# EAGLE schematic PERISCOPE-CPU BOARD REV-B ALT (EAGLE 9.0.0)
This Set of Many Schematics Is what comprises the Revision-B PCB, of my eden project "PERISCOPE". (CPU BOARD ONLY)

## Sheet 1 of 10: Clock, Horizontal Sync
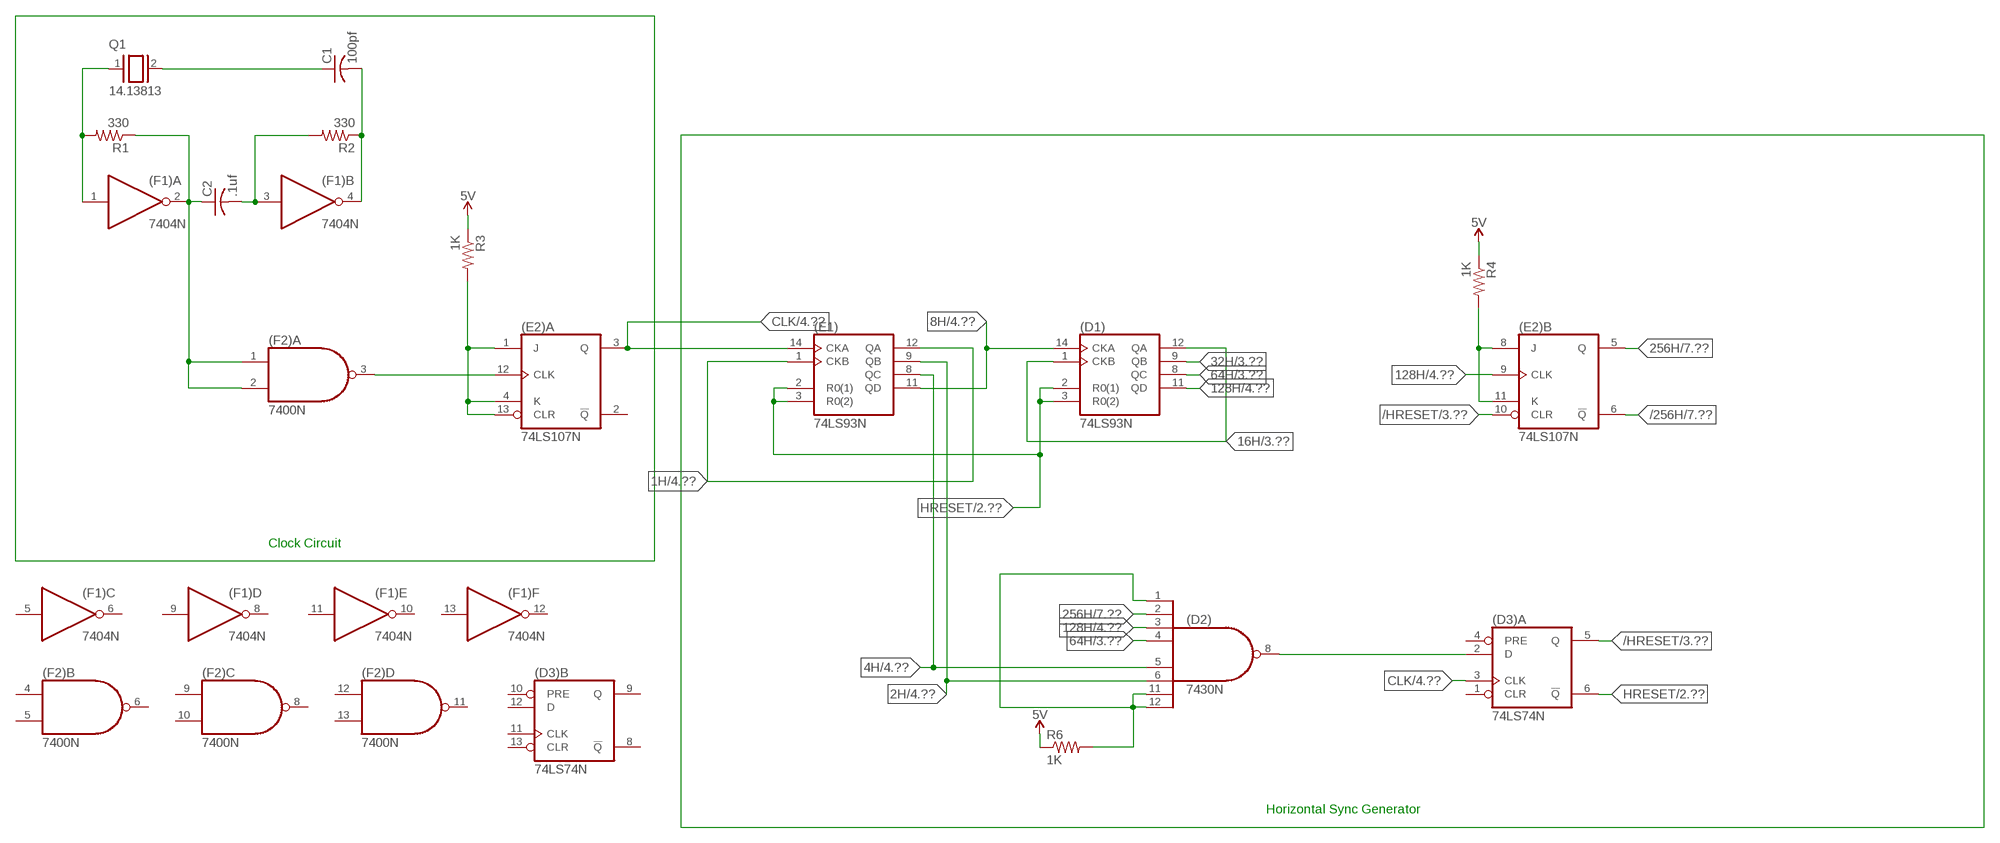
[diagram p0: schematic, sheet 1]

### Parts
(D1)  74LS93N  [DIL14]
(D2)  7430N  [DIL14]
(D3)  74LS74N  [DIL14]
(E1)  74LS93N  [DIL14]
(E2)  74LS107N  [DIL14]
(F1)  7404N  [DIL14]
(F2)  7400N  [DIL14]
C1  100pf  C-US050-025X075  [C050-025X075]
C2  .1uf  C-US050-025X075  [C050-025X075]
Q1  14.13813  XTAL/S  [QS]
R1  330  R-US_0207/10  [0207/10]
R2  330  R-US_0207/10  [0207/10]
R3  1K  R-US_0207/10  [0207/10]
R4  1K  R-US_0207/10  [0207/10]
R6  1K  R-US_0207/10  [0207/10]

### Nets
1H: (E1).1(CKB) (E1).12(QA) ; also sheet 4,8
2H: (D2).6(I5) (E1).9(QB) ; also sheet 4,5,8
4H: (D2).5(I4) (E1).8(QC) ; also sheet 4,7,8
5V: R3.1 R4.1 R6.1 ; also sheet 2
8H: (D1).14(CKA) (E1).11(QD) ; also sheet 4,7,8
16H: (D1).1(CKB) (D1).12(QA) ; also sheet 3,4,7,8
32H: (D1).9(QB) ; also sheet 3,4,7,8
64H: (D1).8(QC) (D2).4(I3) ; also sheet 3,4,7,8
128H: (D1).11(QD) (D2).3(I2) (E2).9(B:CLK) ; also sheet 4,7,8
256H: (D2).2(I1) (E2).5(B:Q) ; also sheet 7,8
512H: (D2).1(I0) (D2).11(I6) (D2).12(I7) R6.2
/256H: (E2).6(B:!Q) ; also sheet 7,8
/HRESET: (D3).5(A:Q) (E2).10(B:CLR) ; also sheet 3,8
CLK: (D3).3(A:CLK) (E1).14(CKA) (E2).3(A:Q) ; also sheet 4,8
HRESET: (D1).2(R0(1)) (D1).3(R0(2)) (D3).6(A:!Q) (E1).2(R0(1)) (E1).3(R0(2)) ; also sheet 2,8
N$1: C1.1 Q1.2
N$2: (F1).4(B:O) C1.2 R2.1
N$3: (F1).2(A:O) (F2).1(A:I0) (F2).2(A:I1) C2.1 R1.1
N$4: (F1).3(B:I) C2.2 R2.2
N$5: (F1).1(A:I) Q1.1 R1.2
N$6: (E2).12(A:CLK) (F2).3(A:O)
N$7: (E2).1(A:J) (E2).4(A:K) (E2).13(A:CLR) R3.2
N$8: (E2).8(B:J) (E2).11(B:K) R4.2
N$11: (D2).8(O) (D3).2(A:D)
Unconnected: (D3).1(A:CLR) (D3).4(A:PRE) (D3).8(B:!Q) (D3).9(B:Q) (D3).10(B:PRE) (D3).11(B:CLK) (D3).12(B:D) (D3).13(B:CLR) (E2).2(A:!Q) (F1).5(C:I) (F1).6(C:O) (F1).8(D:O) (F1).9(D:I) (F1).10(E:O) (F1).11(E:I) (F1).12(F:O) (F1).13(F:I) (F2).4(B:I0) (F2).5(B:I1) (F2).6(B:O) (F2).8(C:O) (F2).9(C:I0) (F2).10(C:I1) (F2).11(D:O) (F2).12(D:I0) (F2).13(D:I1)

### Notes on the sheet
- Clock Circuit
- Horizontal Sync Generator

## Sheet 2 of 10: Vertical Sync Generator
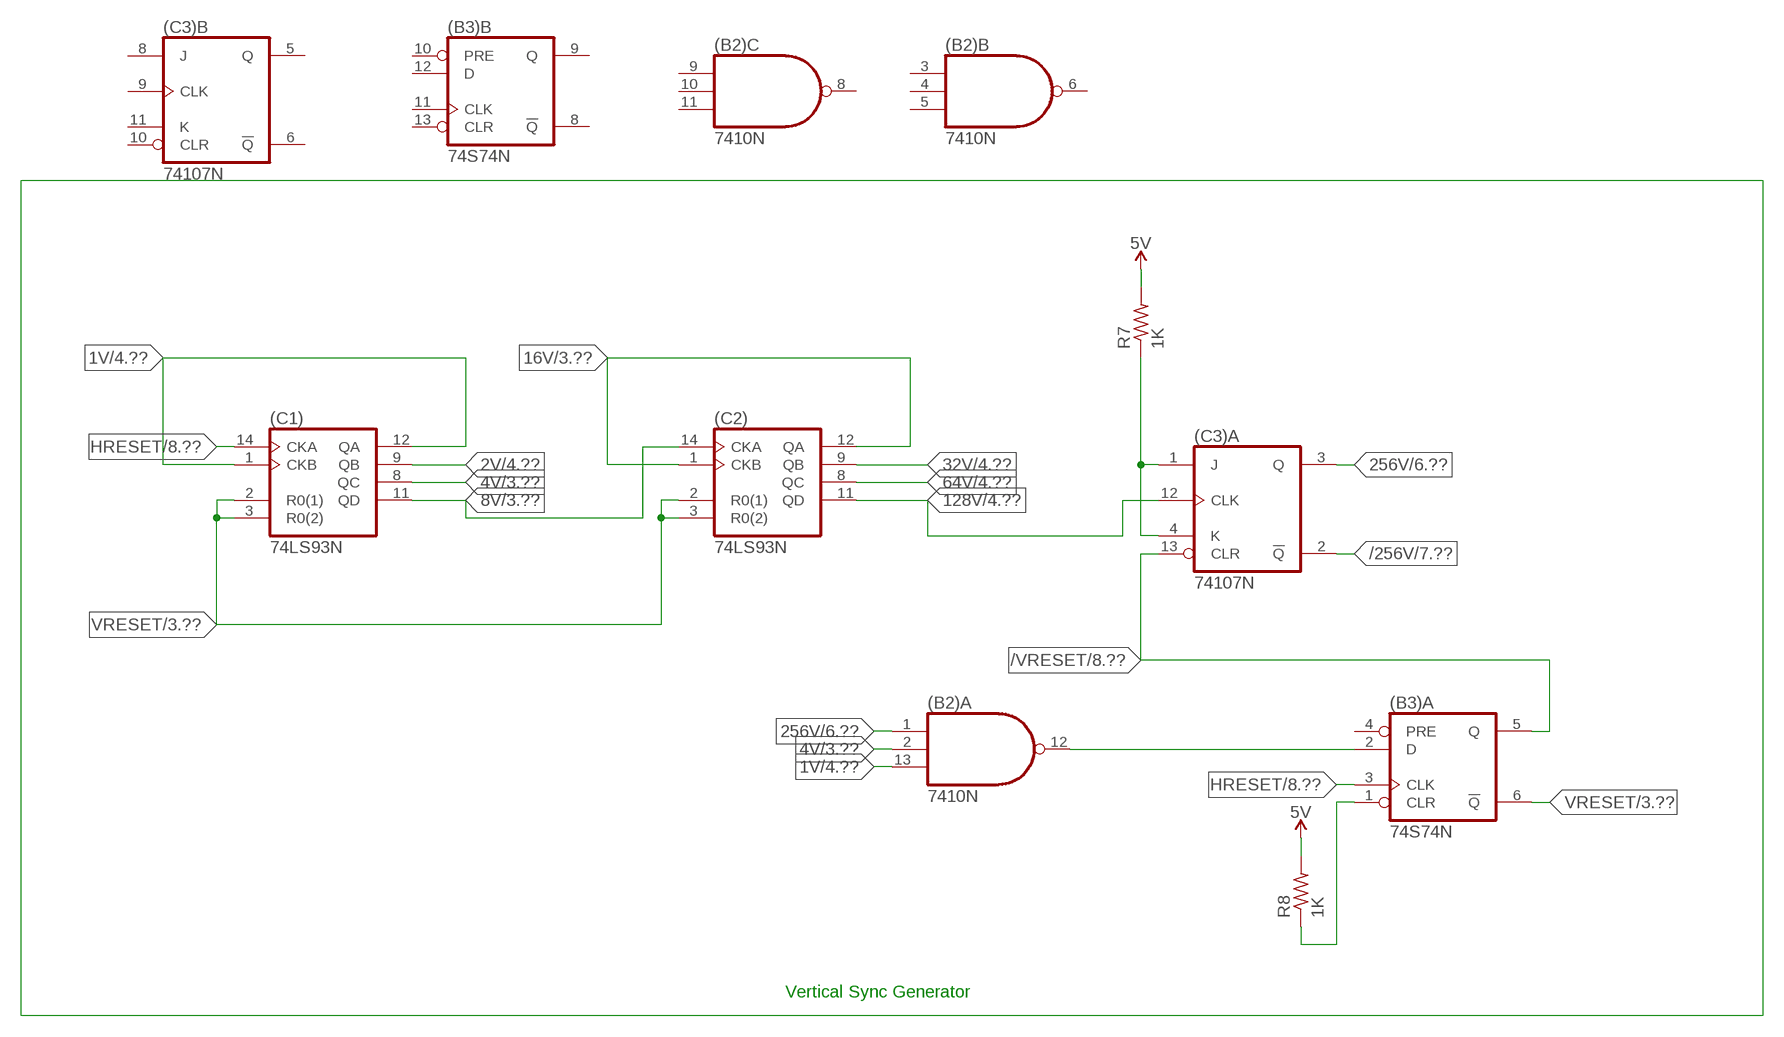
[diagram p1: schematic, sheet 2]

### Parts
(B2)  7410N  [DIL14]
(B3)  74S74N  [DIL14]
(C1)  74LS93N  [DIL14]
(C2)  74LS93N  [DIL14]
(C3)  74107N  [DIL14]
R7  1K  R-US_0207/10  [0207/10]
R8  1K  R-US_0207/10  [0207/10]

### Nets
1V: (B2).13(A:I2) (C1).1(CKB) (C1).12(QA) ; also sheet 4,8
2V: (C1).9(QB) ; also sheet 4,8
4V: (B2).2(A:I1) (C1).8(QC) ; also sheet 3,4,7,8
5V: R7.2 R8.2 ; also sheet 1
8V: (C1).11(QD) (C2).14(CKA) ; also sheet 3,4,7,8
16V: (C2).1(CKB) (C2).12(QA) ; also sheet 3,4,7,8
32V: (C2).9(QB) ; also sheet 4,7,8
64V: (C2).8(QC) ; also sheet 4,8
128V: (C2).11(QD) (C3).12(A:CLK) ; also sheet 4,5,6,8
256V: (B2).1(A:I0) (C3).3(A:Q) ; also sheet 6,8
/256V: (C3).2(A:!Q) ; also sheet 7,8
/VRESET: (B3).5(A:Q) (C3).13(A:CLR) ; also sheet 8
HRESET: (B3).3(A:CLK) (C1).14(CKA) ; also sheet 1,8
N$15: (C3).1(A:J) (C3).4(A:K) R7.1
N$16: (B3).1(A:CLR) R8.1
N$17: (B2).12(A:O) (B3).2(A:D)
VRESET: (B3).6(A:!Q) (C1).2(R0(1)) (C1).3(R0(2)) (C2).2(R0(1)) (C2).3(R0(2)) ; also sheet 3,8
Unconnected: (B2).3(B:I0) (B2).4(B:I1) (B2).5(B:I2) (B2).6(B:O) (B2).8(C:O) (B2).9(C:I0) (B2).10(C:I1) (B2).11(C:I2) (B3).4(A:PRE) (B3).8(B:!Q) (B3).9(B:Q) (B3).10(B:PRE) (B3).11(B:CLK) (B3).12(B:D) (B3).13(B:CLR) (C3).5(B:Q) (C3).6(B:!Q) (C3).8(B:J) (C3).9(B:CLK) (C3).10(B:CLR) (C3).11(B:K)

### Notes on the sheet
- Vertical Sync Generator

## Sheet 3 of 10: Sync Generation
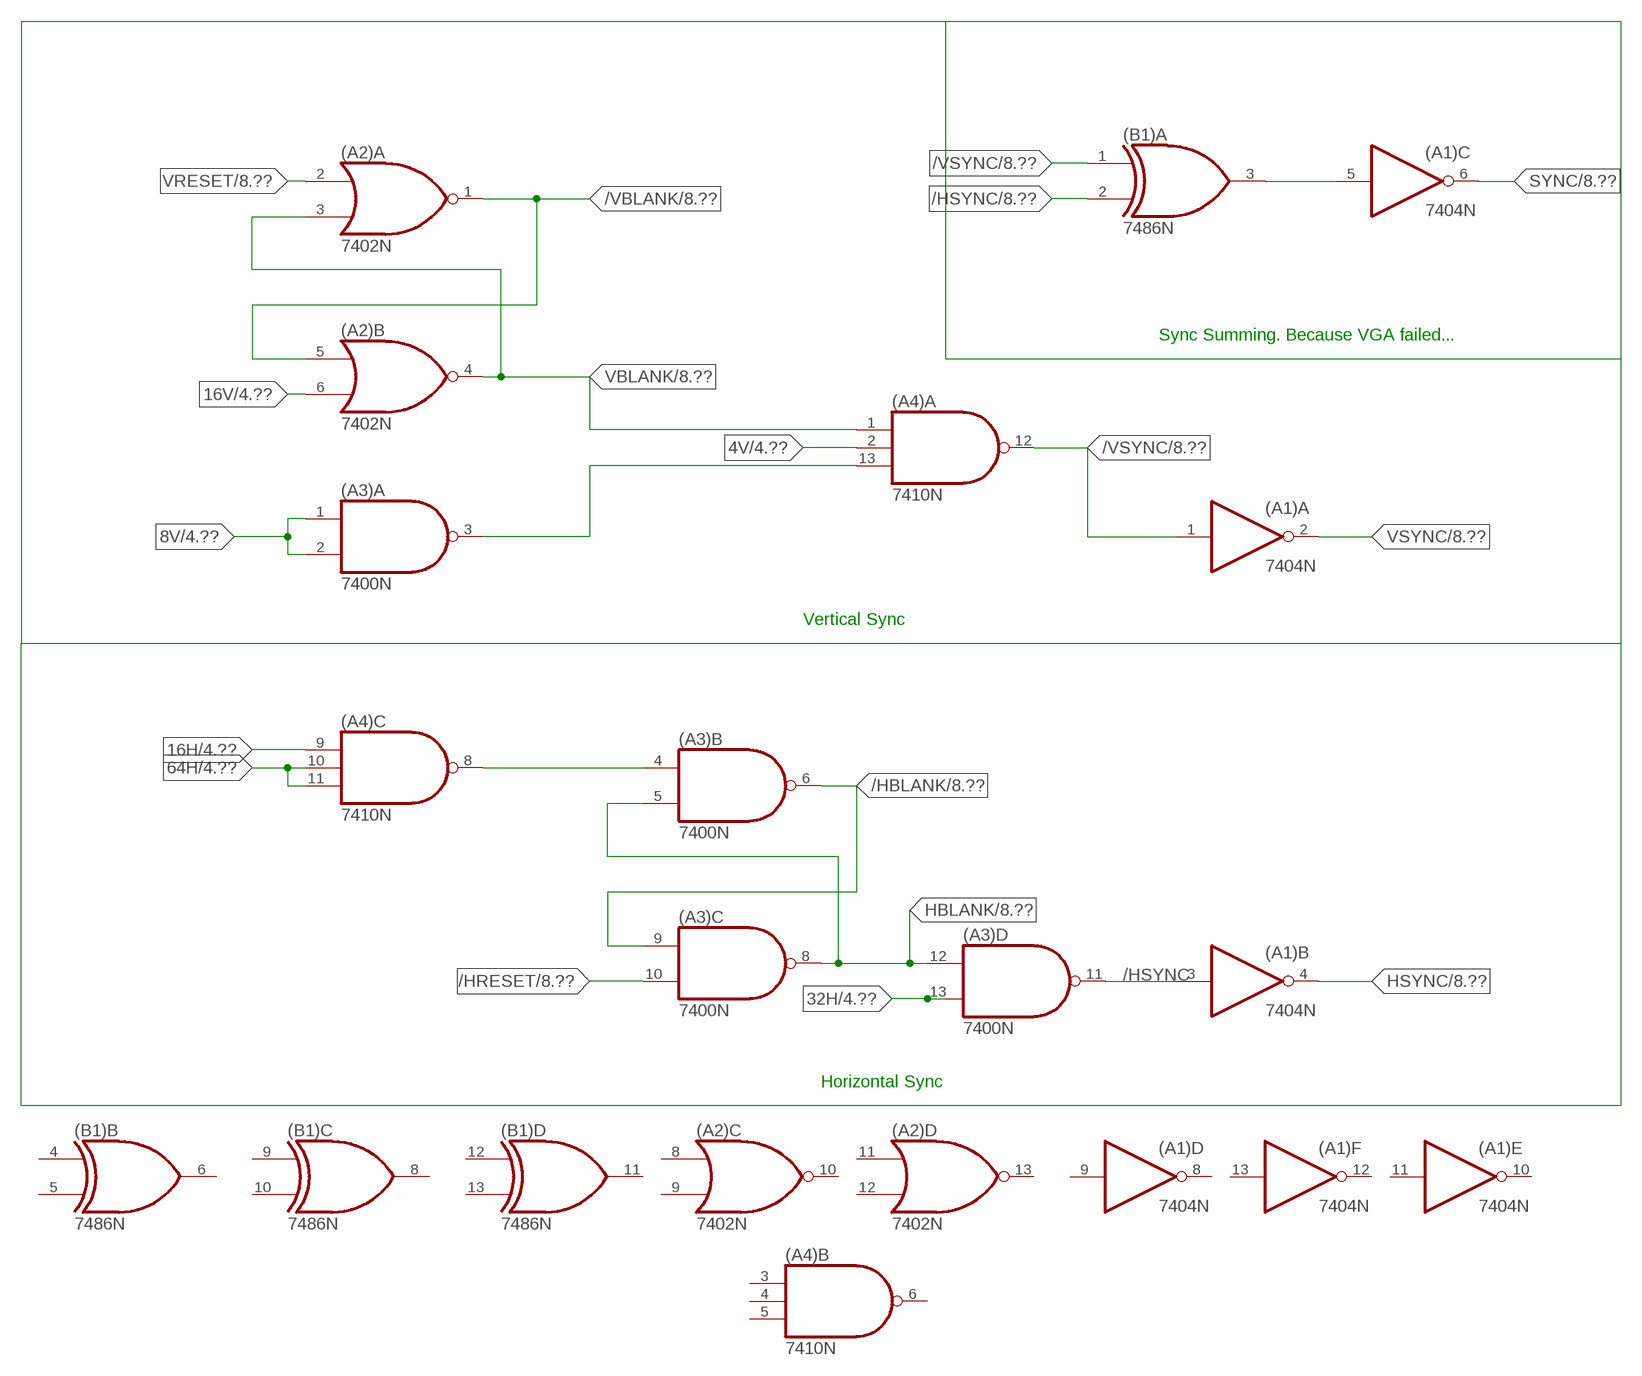
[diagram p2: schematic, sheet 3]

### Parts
(A1)  7404N  [DIL14]
(A2)  7402N  [DIL14]
(A3)  7400N  [DIL14]
(A4)  7410N  [DIL14]
(B1)  7486N  [DIL14]

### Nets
4V: (A4).2(A:I1) ; also sheet 2,4,7,8
8V: (A3).1(A:I0) (A3).2(A:I1) ; also sheet 2,4,7,8
16H: (A4).9(C:I0) ; also sheet 1,4,7,8
16V: (A2).6(B:I1) ; also sheet 2,4,7,8
32H: (A3).13(D:I1) ; also sheet 1,4,7,8
64H: (A4).10(C:I1) (A4).11(C:I2) ; also sheet 1,4,7,8
/HBLANK: (A3).6(B:O) (A3).9(C:I0) ; also sheet 8
/HRESET: (A3).10(C:I1) ; also sheet 1,8
/HSYNC: (A1).3(B:I) (A3).11(D:O) (B1).2(A:I1) ; also sheet 8
/VBLANK: (A2).1(A:O) (A2).5(B:I0) ; also sheet 8
/VSYNC: (A1).1(A:I) (A4).12(A:O) (B1).1(A:I0) ; also sheet 8
HBLANK: (A3).5(B:I1) (A3).8(C:O) (A3).12(D:I0) ; also sheet 8
HSYNC: (A1).4(B:O) ; also sheet 8
N$19: (A3).4(B:I0) (A4).8(C:O)
N$20: (A3).3(A:O) (A4).13(A:I2)
N$22: (A1).5(C:I) (B1).3(A:O)
SYNC: (A1).6(C:O) ; also sheet 8,10
VBLANK: (A2).3(A:I1) (A2).4(B:O) (A4).1(A:I0) ; also sheet 8
VRESET: (A2).2(A:I0) ; also sheet 2,8
VSYNC: (A1).2(A:O) ; also sheet 8
Unconnected: (A1).8(D:O) (A1).9(D:I) (A1).10(E:O) (A1).11(E:I) (A1).12(F:O) (A1).13(F:I) (A2).8(C:I0) (A2).9(C:I1) (A2).10(C:O) (A2).11(D:I0) (A2).12(D:I1) (A2).13(D:O) (A4).3(B:I0) (A4).4(B:I1) (A4).5(B:I2) (A4).6(B:O) (B1).4(B:I0) (B1).5(B:I1) (B1).6(B:O) (B1).8(C:O) (B1).9(C:I0) (B1).10(C:I1) (B1).11(D:O) (B1).12(D:I0) (B1).13(D:I1)

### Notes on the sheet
- Sync Summing. Because VGA failed...
- Vertical Sync
- Horizontal Sync

## Sheet 4 of 10: SYNC INVERSION
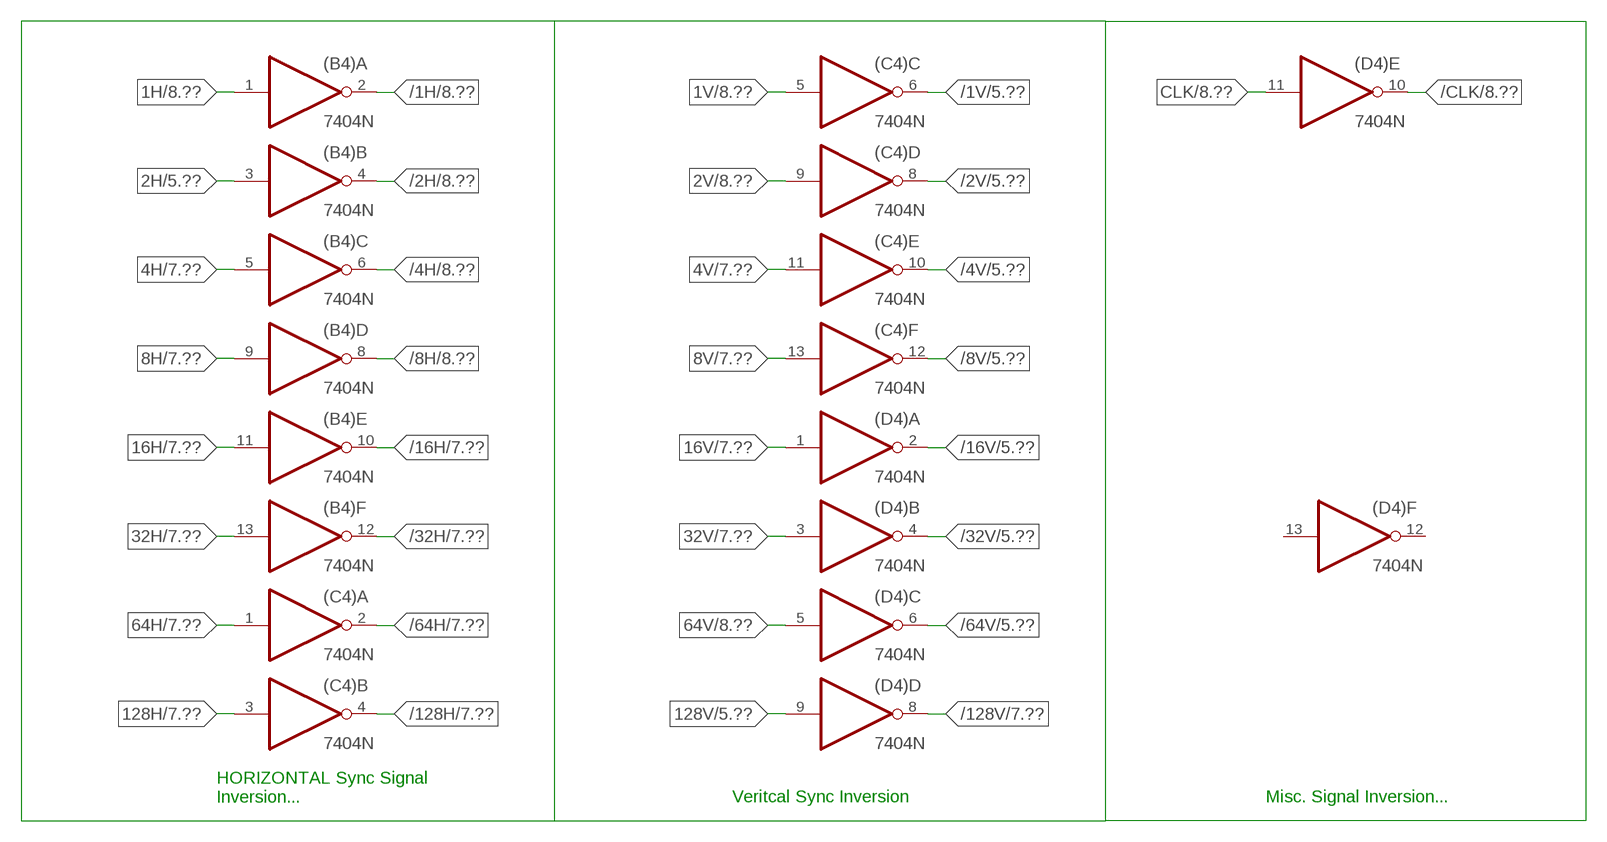
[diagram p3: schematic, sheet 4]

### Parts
(B4)  7404N  [DIL14]
(C4)  7404N  [DIL14]
(D4)  7404N  [DIL14]

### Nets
1H: (B4).1(A:I) ; also sheet 1,8
1V: (C4).5(C:I) ; also sheet 2,8
2H: (B4).3(B:I) ; also sheet 1,5,8
2V: (C4).9(D:I) ; also sheet 2,8
4H: (B4).5(C:I) ; also sheet 1,7,8
4V: (C4).11(E:I) ; also sheet 2,3,7,8
8H: (B4).9(D:I) ; also sheet 1,7,8
8V: (C4).13(F:I) ; also sheet 2,3,7,8
16H: (B4).11(E:I) ; also sheet 1,3,7,8
16V: (D4).1(A:I) ; also sheet 2,3,7,8
32H: (B4).13(F:I) ; also sheet 1,3,7,8
32V: (D4).3(B:I) ; also sheet 2,7,8
64H: (C4).1(A:I) ; also sheet 1,3,7,8
64V: (D4).5(C:I) ; also sheet 2,8
128H: (C4).3(B:I) ; also sheet 1,7,8
128V: (D4).9(D:I) ; also sheet 2,5,6,8
/1H: (B4).2(A:O) ; also sheet 8
/1V: (C4).6(C:O) ; also sheet 5,8
/2H: (B4).4(B:O) ; also sheet 8
/2V: (C4).8(D:O) ; also sheet 5,8
/4H: (B4).6(C:O) ; also sheet 8
/4V: (C4).10(E:O) ; also sheet 5,8
/8H: (B4).8(D:O) ; also sheet 8
/8V: (C4).12(F:O) ; also sheet 5,8
/16H: (B4).10(E:O) ; also sheet 7,8
/16V: (D4).2(A:O) ; also sheet 5,7,8
/32H: (B4).12(F:O) ; also sheet 7,8
/32V: (D4).4(B:O) ; also sheet 5,8
/64H: (C4).2(A:O) ; also sheet 7,8
/64V: (D4).6(C:O) ; also sheet 5,7,8
/128H: (C4).4(B:O) ; also sheet 7,8
/128V: (D4).8(D:O) ; also sheet 7,8
/CLK: (D4).10(E:O) ; also sheet 8
CLK: (D4).11(E:I) ; also sheet 1,8
Unconnected: (D4).12(F:O) (D4).13(F:I)

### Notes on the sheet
- HORIZONTAL Sync Signal
  Inversion...
- Veritcal Sync Inversion | Misc. Signal Inversion...

## Sheet 5 of 10: Ocean Generation, Surface and Floor
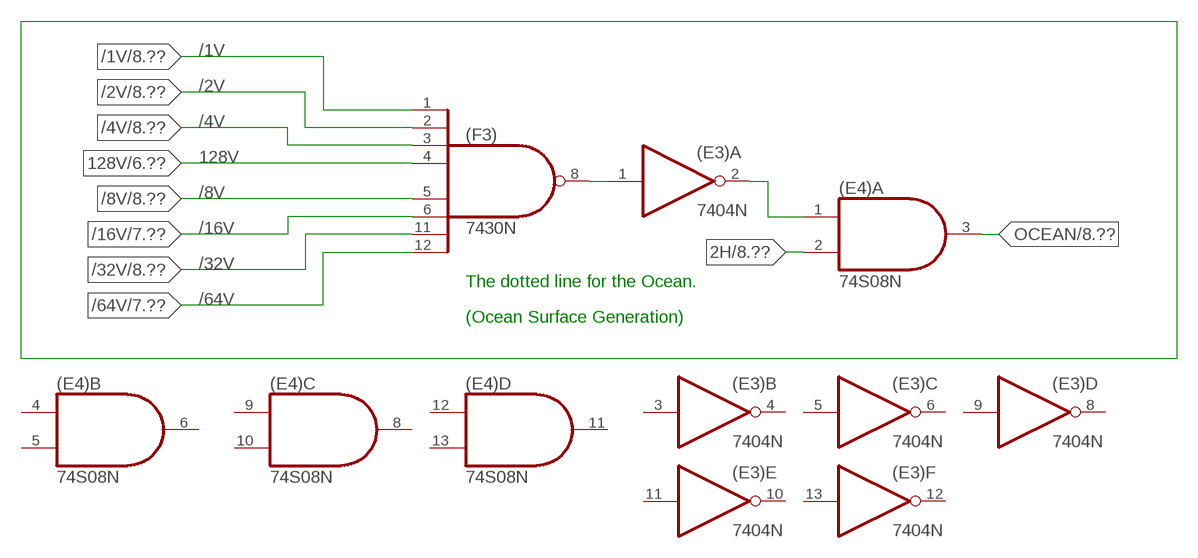
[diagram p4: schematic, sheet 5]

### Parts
(E3)  7404N  [DIL14]
(E4)  74S08N  [DIL14]
(F3)  7430N  [DIL14]

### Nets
2H: (E4).2(A:I1) ; also sheet 1,4,8
128V: (F3).4(I3) ; also sheet 2,4,6,8
/1V: (F3).1(I0) ; also sheet 4,8
/2V: (F3).2(I1) ; also sheet 4,8
/4V: (F3).3(I2) ; also sheet 4,8
/8V: (F3).5(I4) ; also sheet 4,8
/16V: (F3).6(I5) ; also sheet 4,7,8
/32V: (F3).11(I6) ; also sheet 4,8
/64V: (F3).12(I7) ; also sheet 4,7,8
N$28: (E3).1(A:I) (F3).8(O)
N$29: (E3).2(A:O) (E4).1(A:I0)
OCEAN: (E4).3(A:O) ; also sheet 8,9
Unconnected: (E3).3(B:I) (E3).4(B:O) (E3).5(C:I) (E3).6(C:O) (E3).8(D:O) (E3).9(D:I) (E3).10(E:O) (E3).11(E:I) (E3).12(F:O) (E3).13(F:I) (E4).4(B:I0) (E4).5(B:I1) (E4).6(B:O) (E4).8(C:O) (E4).9(C:I0) (E4).10(C:I1) (E4).11(D:O) (E4).12(D:I0) (E4).13(D:I1)

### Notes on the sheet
- The dotted line for the Ocean.
- (Ocean Surface Generation)

## Sheet 6 of 10: Coin Circuitry
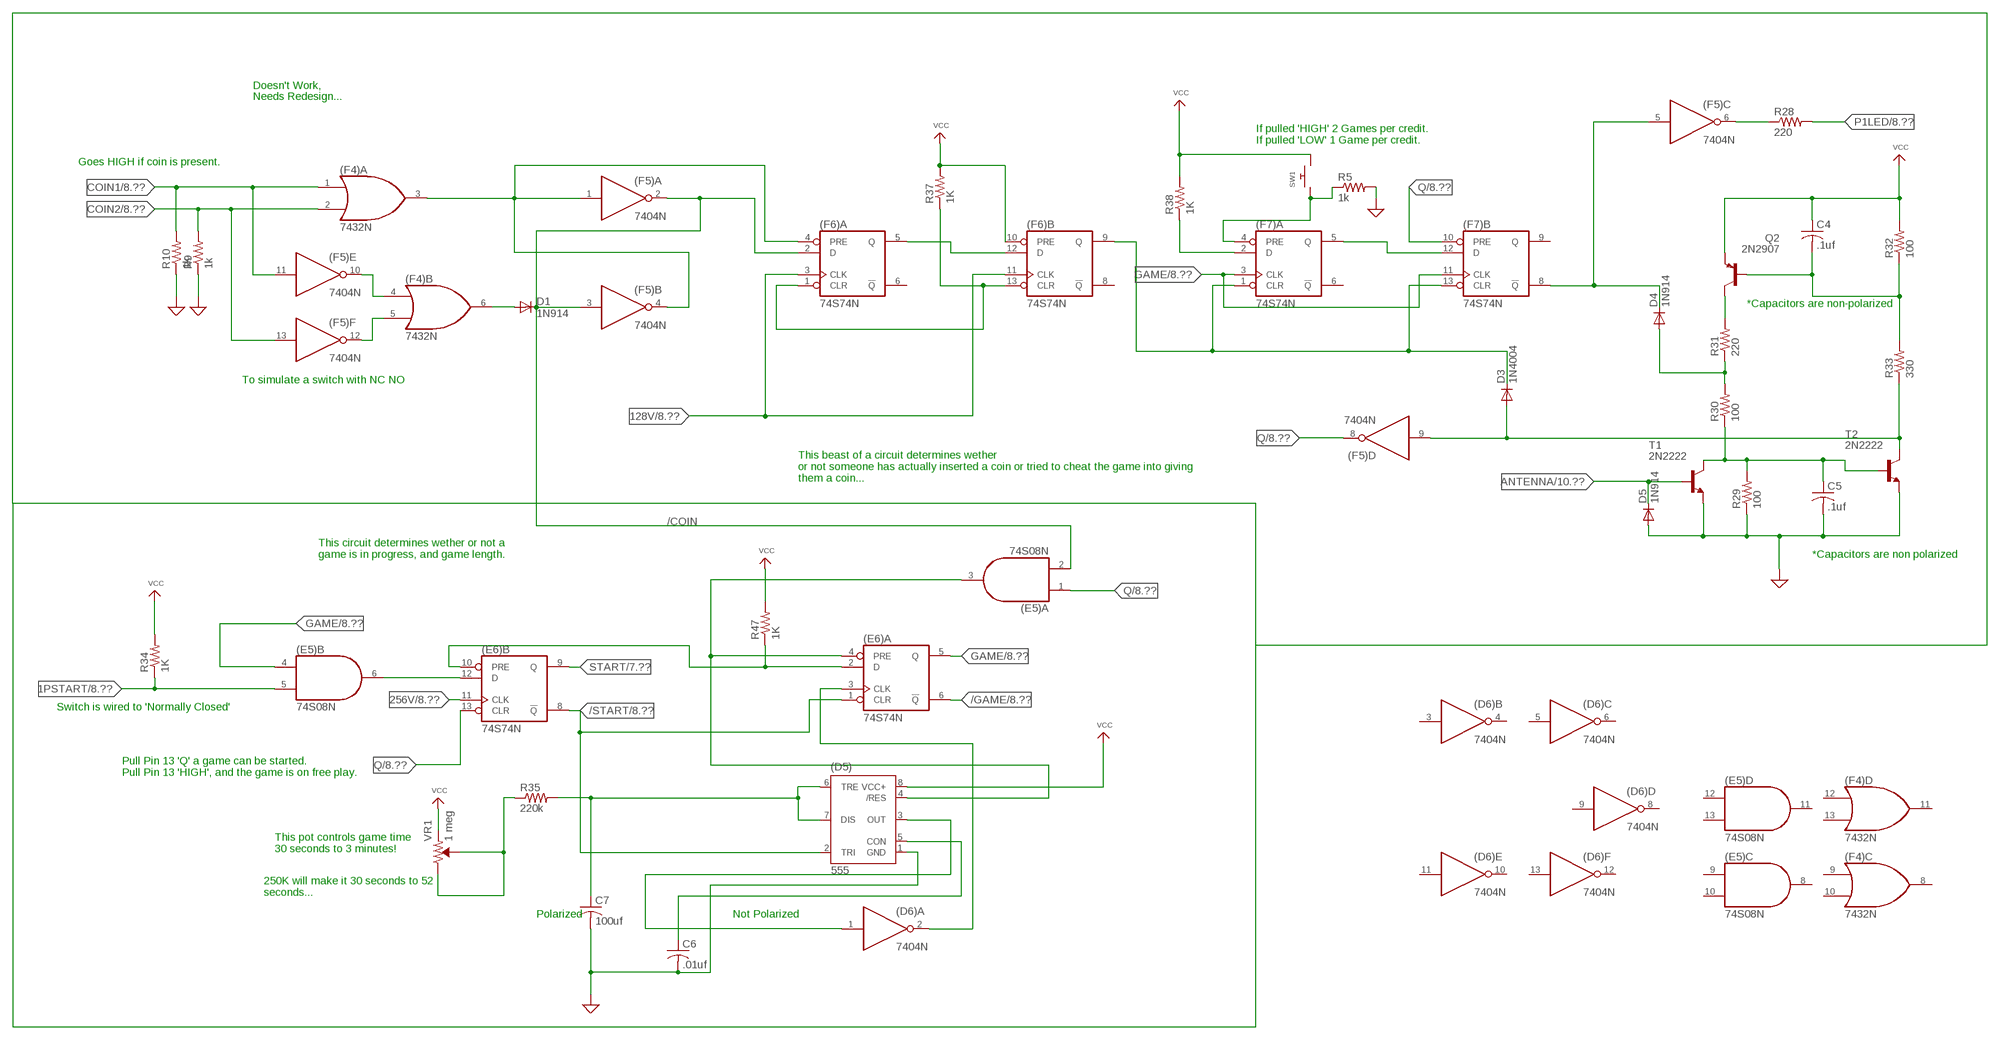
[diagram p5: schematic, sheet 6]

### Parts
(D5)  555  555P  [DIP08]
(D6)  7404N  [DIL14]
(E5)  74S08N  [DIL14]
(E6)  74S74N  [DIL14]
(F4)  7432N  [DIL14]
(F5)  7404N  [DIL14]
(F6)  74S74N  [DIL14]
(F7)  74S74N  [DIL14]
C4  .1uf  C-US025-024X044  [C025-024X044]
C5  .1uf  C-US025-024X044  [C025-024X044]
C6  .01uf  C-US025-024X044  [C025-024X044]
C7  100uf  C-US025-024X044  [C025-024X044]
D1  1N914  1N4004  [DO41-10]
D3  1N4004  [DO41-10]
D4  1N914  1N4004  [DO41-10]
D5  1N914  1N4004  [DO41-10]
Q2  2N2907  [TO92-EBC-OVAL]
R5  1k  R-US_0207/10  [0207/10]
R9  1k  R-US_0207/10  [0207/10]
R10  1k  R-US_0207/10  [0207/10]
R28  220  R-US_0207/10  [0207/10]
R29  100  R-US_0207/10  [0207/10]
R30  100  R-US_0207/10  [0207/10]
R31  220  R-US_0207/10  [0207/10]
R32  100  R-US_0207/10  [0207/10]
R33  330  R-US_0207/10  [0207/10]
R34  1K  R-US_0207/10  [0207/10]
R35  220k  R-US_0207/10  [0207/10]
R37  1K  R-US_0207/10  [0207/10]
R38  1K  R-US_0207/10  [0207/10]
R47  1K  R-US_0207/10  [0207/10]
SW1  SWITCH_PUSHBUTTONEVQ-PE  [TACT_PANA-EVQ]
T1  2N2222  [TO92-EBC-OVAL]
T2  2N2222  [TO92-EBC-OVAL]
VR1  1 meg  TRIMPOT-PTH-10MM-KNOB-1/2W-10%  [TRIMPOT-PTH-3386U]

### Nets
1PSTART: (E5).5(B:I1) R34.1 ; also sheet 8,10
128V: (F6).3(A:CLK) (F6).11(B:CLK) ; also sheet 2,4,5,8
256V: (E6).11(B:CLK) ; also sheet 2,8
/COIN: (E5).2(A:I1) (F5).2(A:O) (F5).3(B:I) (F6).2(A:D) D1.C
/GAME: (E6).6(A:!Q) ; also sheet 8
/START: (D5).2(TRI) (E6).1(A:CLR) (E6).8(B:!Q) ; also sheet 8
ANTENNA: D5.C T1.B ; also sheet 10
COIN1: (F4).1(A:I0) (F5).11(E:I) R10.2 ; also sheet 8,10
COIN2: (F4).2(A:I1) (F5).13(F:I) R9.2 ; also sheet 8,10
GAME: (E5).4(B:I0) (E6).5(A:Q) (F7).3(A:CLK) (F7).11(B:CLK) ; also sheet 8
GND: (D5).1(GND) C5.2 C6.2 C7.2 D5.A R5.2 R9.1 R10.1 R29.1 T1.E T2.E ; supply symbol labelled SUP ; also sheet 7,9,10
N$38: (F4).4(B:I0) (F5).10(E:O)
N$39: (F4).5(B:I1) (F5).12(F:O)
N$95: Q2.C R31.2
N$96: (F7).5(A:Q) (F7).12(B:D)
N$97: (F6).5(A:Q) (F6).12(B:D)
N$98: (F4).3(A:O) (F5).1(A:I) (F5).4(B:O) (F6).4(A:PRE)
N$99: (F6).9(B:Q) (F7).1(A:CLR) (F7).13(B:CLR) D3.C
N$100: (F7).4(A:PRE) R5.1 SW1.P$1
N$101: (F5).5(C:I) (F7).8(B:!Q) D4.C
N$102: (F5).6(C:O) R28.1
N$103: D4.A R30.2 R31.1
N$104: (D5).4(/RES) (E5).3(A:O) (E6).4(A:PRE)
N$105: (F5).9(D:I) D3.A R33.1 T2.C
N$106: C4.2 Q2.B R32.1 R33.2
N$107: C5.1 R29.2 R30.1 T1.C T2.B
N$108: (E5).6(B:O) (E6).12(B:D)
N$109: (D5).5(CON) C6.1
N$112: (D6).2(A:O) (E6).3(A:CLK)
N$114: (D5).3(OUT) (D6).1(A:I)
N$116: (D5).6(TRE) (D5).7(DIS) C7.1 R35.2
N$118: R35.1 VR1.2(WIPER) VR1.3(CW)
N$119: (F4).6(B:O) D1.A
N$120: (F6).1(A:CLR) (F6).13(B:CLR) R37.1
N$123: (F7).2(A:D) R38.1
N$213: (E6).2(A:D) (E6).10(B:PRE) R47.1
P1LED: R28.2 ; also sheet 8,10
Q: (E5).1(A:I0) (E6).13(B:CLR) (F5).8(D:O) (F7).10(B:PRE) ; also sheet 8
START: (E6).9(B:Q) ; also sheet 7,8
VCC: (D5).8(VCC+) (F6).10(B:PRE) C4.1 Q2.E R32.2 R34.2 R37.2 R38.2 R47.2 SW1.P$2 VR1.1(CCW) ; also sheet 7,10
Unconnected: (D6).3(B:I) (D6).4(B:O) (D6).5(C:I) (D6).6(C:O) (D6).8(D:O) (D6).9(D:I) (D6).10(E:O) (D6).11(E:I) (D6).12(F:O) (D6).13(F:I) (E5).8(C:O) (E5).9(C:I0) (E5).10(C:I1) (E5).11(D:O) (E5).12(D:I0) (E5).13(D:I1) (F4).8(C:O) (F4).9(C:I0) (F4).10(C:I1) (F4).11(D:O) (F4).12(D:I0) (F4).13(D:I1) (F6).6(A:!Q) (F6).8(B:!Q) (F7).6(A:!Q) (F7).9(B:Q)

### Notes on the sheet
- Doesn't Work,
- Needs Redesign...
- If pulled 'HIGH' 2 Games per credit.
  If pulled 'LOW' 1 Game per credit.
- Goes HIGH if coin is present.
- *Capacitors are non-polarized
- To simulate a switch with NC NO
- This beast of a circuit determines wether 
  or not someone has actually inserted a coin or tried to cheat the game into giving
  them a coin...
- This circuit determines wether or not a
  game is in progress, and game length.
- *Capacitors are non polarized
- Switch is wired to 'Normally Closed'
- Pull Pin 13 'Q' a game can be started.
  Pull Pin 13 'HIGH', and the game is on free play.
- This pot controls game time
  30 seconds to 3 minutes!
- 250K will make it 30 seconds to 52
  seconds...
- Polarized | Not Polarized

## Sheet 7 of 10: Score
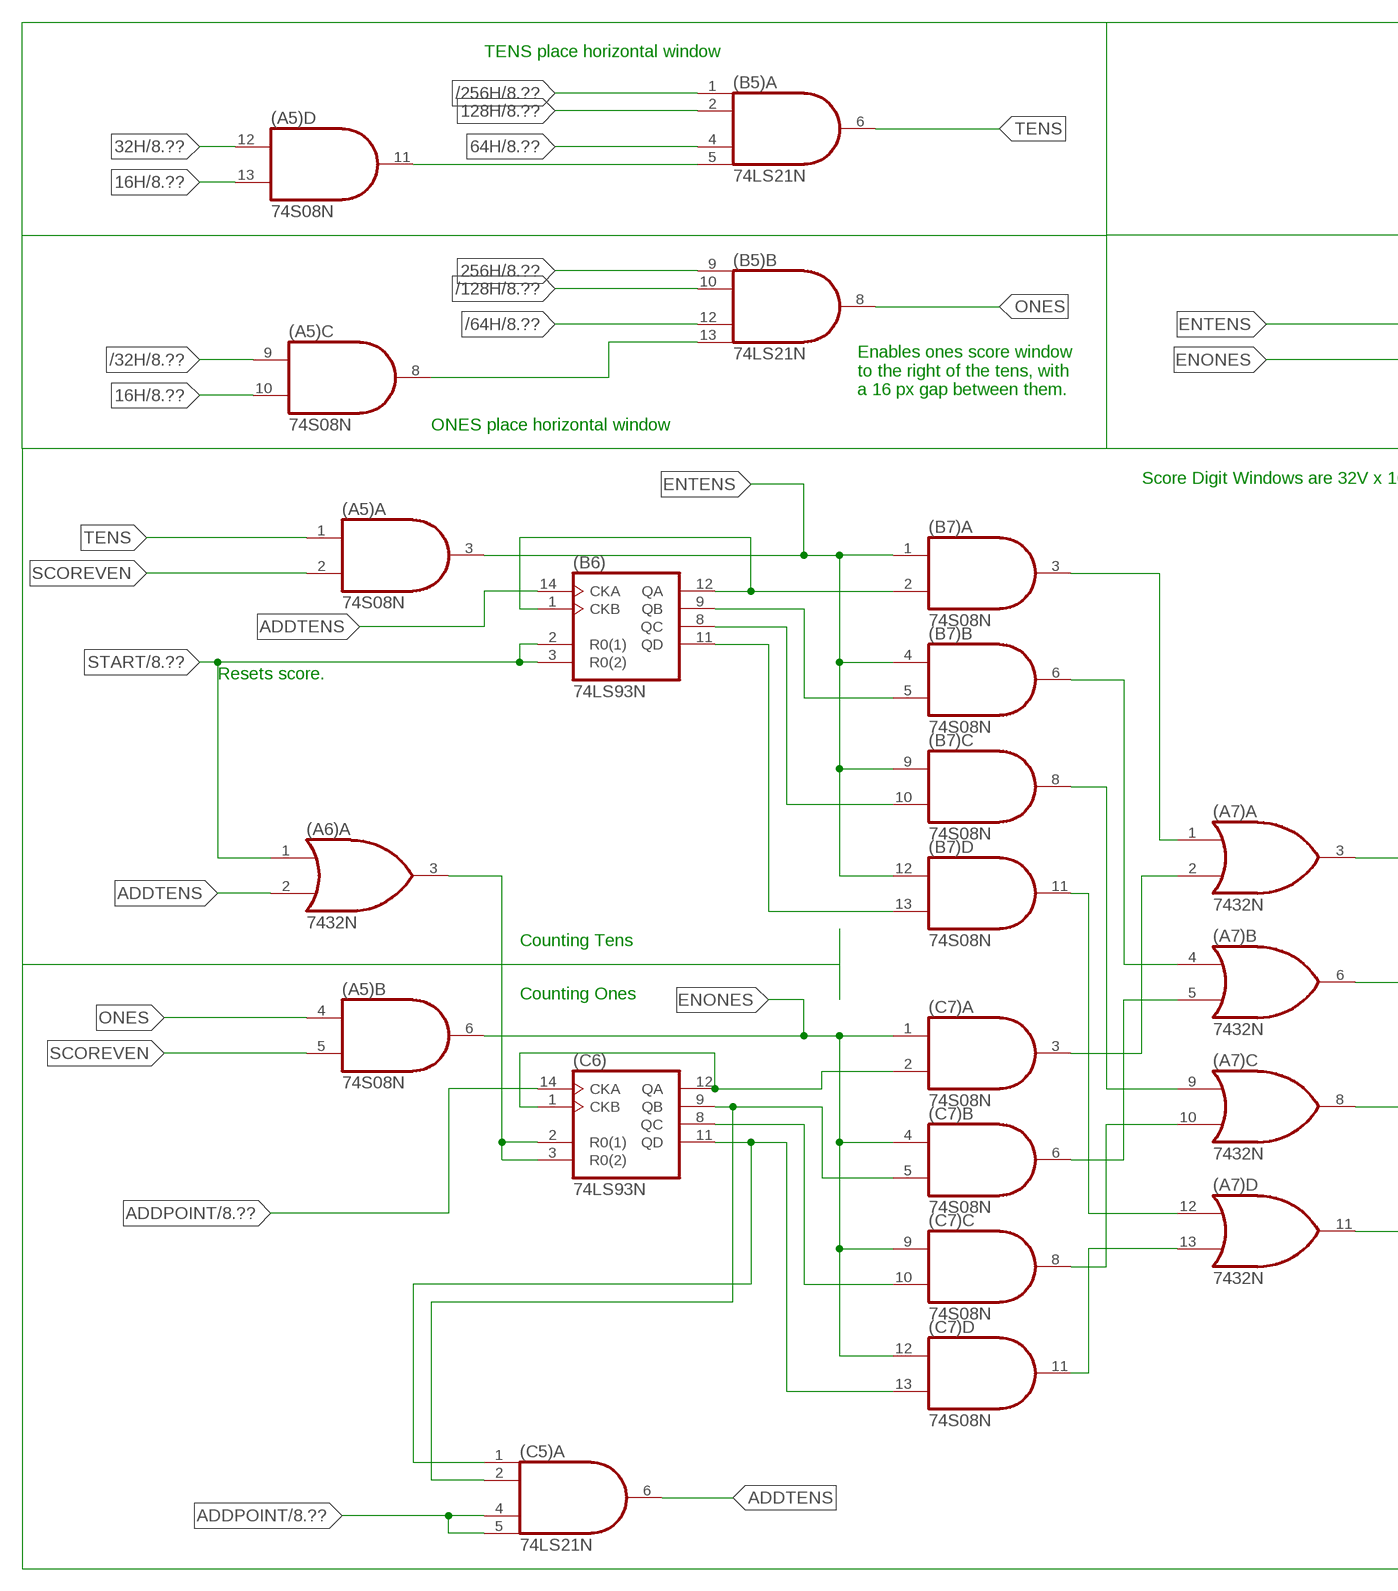
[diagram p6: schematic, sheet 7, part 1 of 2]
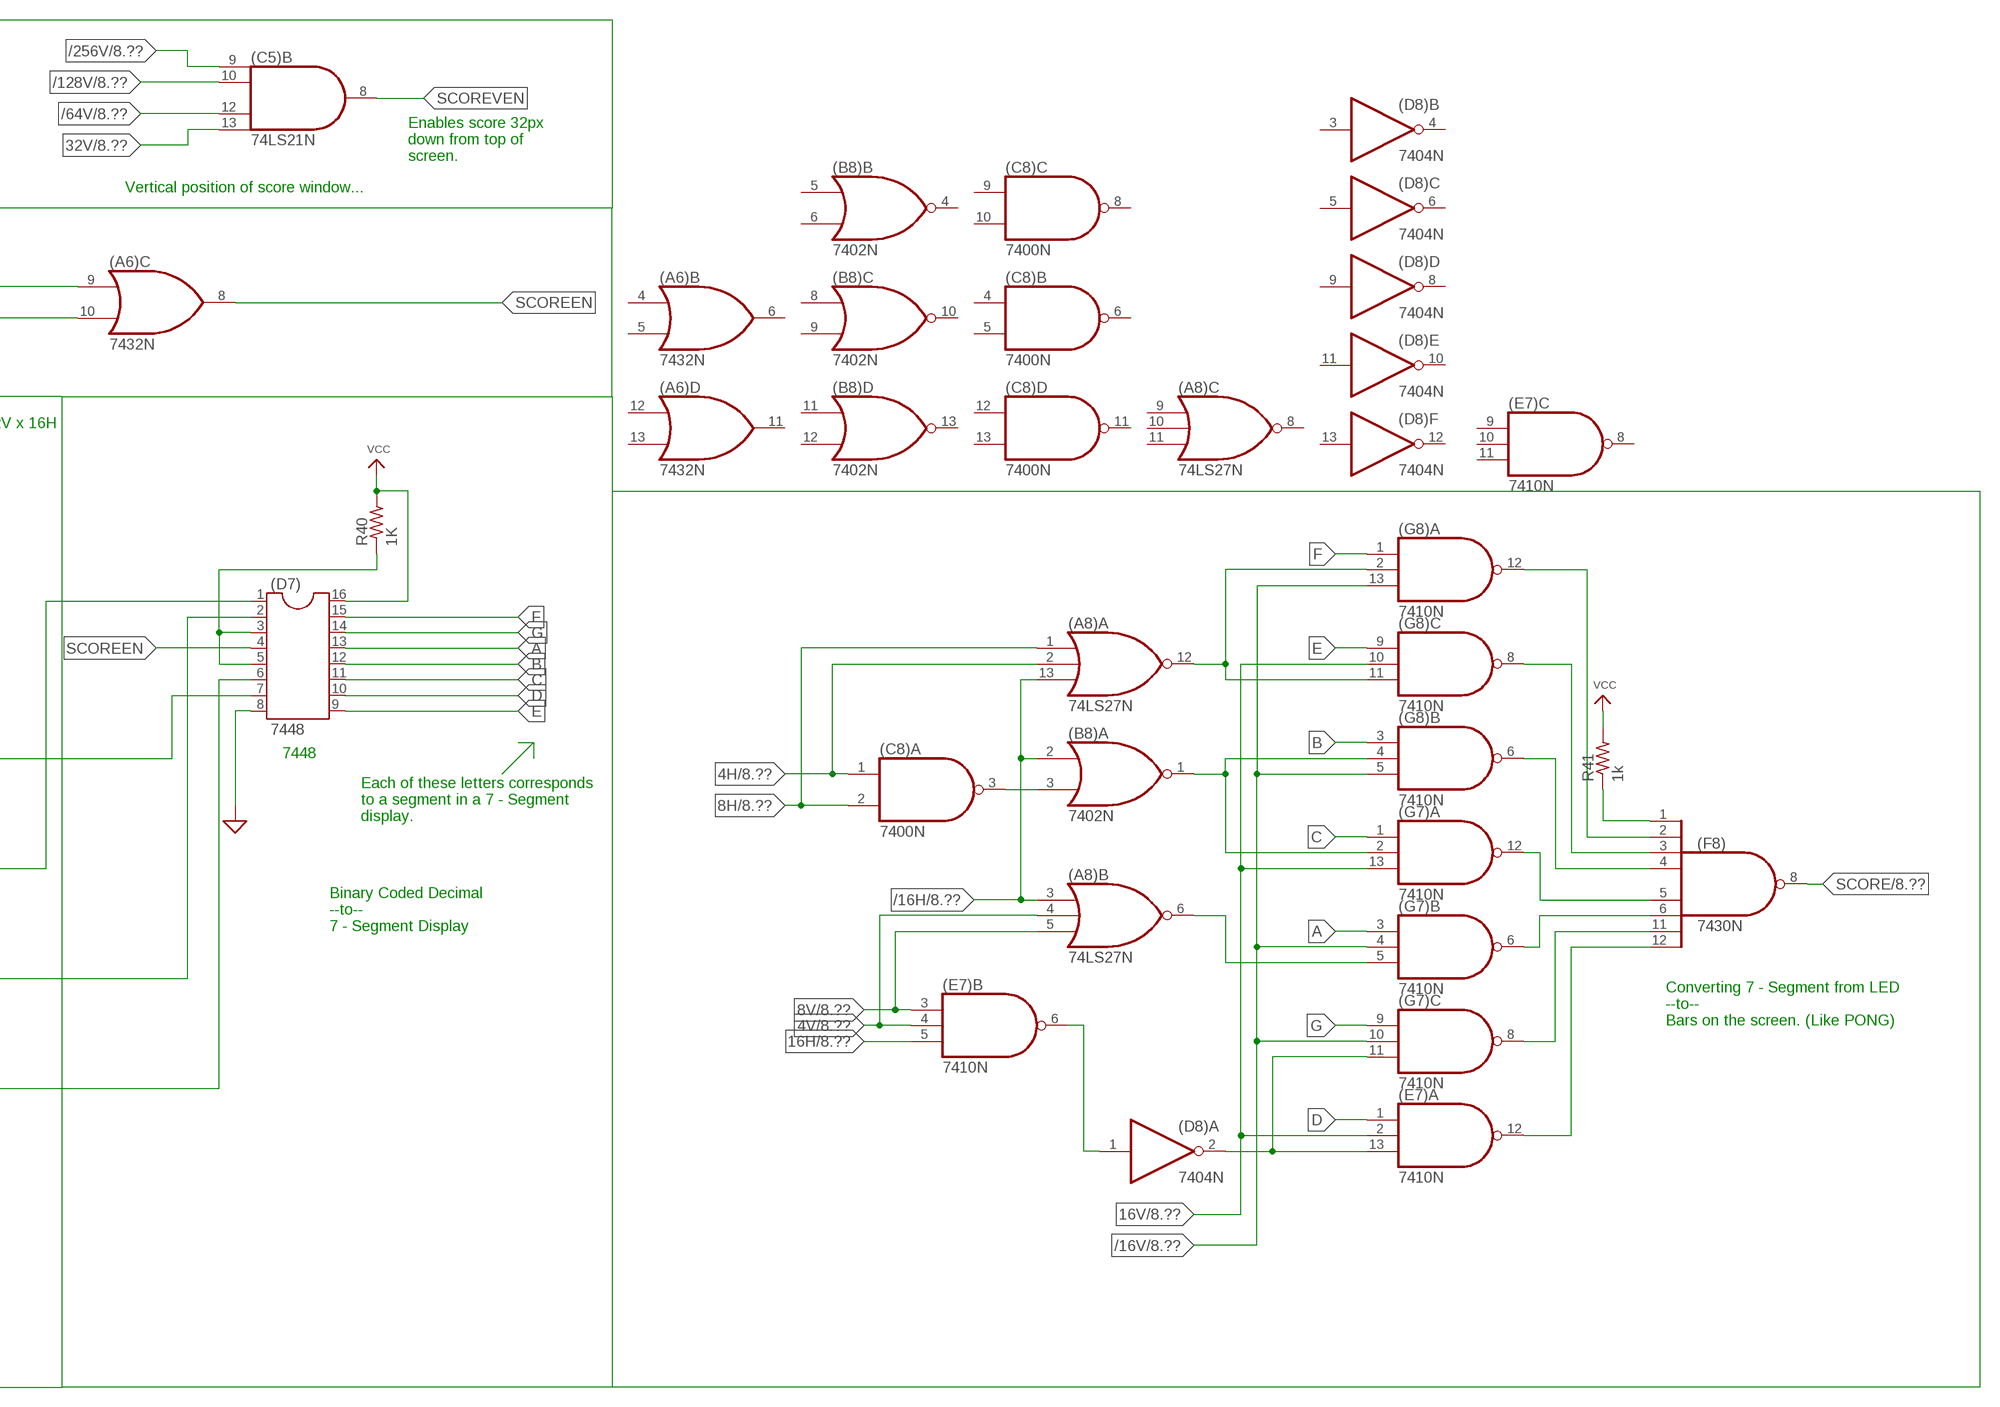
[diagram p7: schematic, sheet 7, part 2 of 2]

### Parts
(A5)  74S08N  [DIL14]
(A6)  7432N  [DIL14]
(A7)  7432N  [DIL14]
(A8)  74LS27N  [DIL14]
(B5)  74LS21N  [DIL14]
(B6)  74LS93N  [DIL14]
(B7)  74S08N  [DIL14]
(B8)  7402N  [DIL14]
(C5)  74LS21N  [DIL14]
(C6)  74LS93N  [DIL14]
(C7)  74S08N  [DIL14]
(C8)  7400N  [DIL14]
(D7)  7448  DIL16S  [SOCKET-16]
(D8)  7404N  [DIL14]
(E7)  7410N  [DIL14]
(F8)  7430N  [DIL14]
(G7)  7410N  [DIL14]
(G8)  7410N  [DIL14]
R40  1K  R-US_0207/10  [0207/10]
R41  1k  R-US_0207/10  [0207/10]

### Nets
4H: (A8).2(A:I1) (C8).1(A:I0) ; also sheet 1,4,8
4V: (A8).4(B:I1) (E7).4(B:I1) ; also sheet 2,3,4,8
8H: (A8).1(A:I0) (C8).2(A:I1) ; also sheet 1,4,8
8V: (A8).5(B:I2) (E7).3(B:I0) ; also sheet 2,3,4,8
16H: (A5).10(C:I1) (A5).13(D:I1) (E7).5(B:I2) ; also sheet 1,3,4,8
16V: (E7).2(A:I1) (G7).13(A:I2) (G8).10(C:I1) ; also sheet 2,3,4,8
32H: (A5).12(D:I0) ; also sheet 1,3,4,8
32V: (C5).13(B:I3) ; also sheet 2,4,8
64H: (B5).4(A:I2) ; also sheet 1,3,4,8
128H: (B5).2(A:I1) ; also sheet 1,4,8
256H: (B5).9(B:I0) ; also sheet 1,8
/16H: (A8).3(B:I0) (A8).13(A:I2) (B8).2(A:I0) ; also sheet 4,8
/16V: (G7).4(B:I1) (G7).10(C:I1) (G8).5(B:I2) (G8).13(A:I2) ; also sheet 4,5,8
/32H: (A5).9(C:I0) ; also sheet 4,8
/64H: (B5).12(B:I2) ; also sheet 4,8
/64V: (C5).12(B:I2) ; also sheet 4,5,8
/128H: (B5).10(B:I1) ; also sheet 4,8
/128V: (C5).10(B:I1) ; also sheet 4,8
/256H: (B5).1(A:I0) ; also sheet 1,8
/256V: (C5).9(B:I0) ; also sheet 2,8
A: (D7).13 (G7).3(B:I0)
ADDPOINT: (C5).4(A:I2) (C5).5(A:I3) (C6).14(CKA) ; also sheet 8
ADDTENS: (A6).2(A:I1) (B6).14(CKA) (C5).6(A:O)
B: (D7).12 (G8).3(B:I0)
C: (D7).11 (G7).1(A:I0)
D: (D7).10 (E7).1(A:I0)
E: (D7).9 (G8).9(C:I0)
ENONES: (A5).6(B:O) (A6).10(C:I1) (C7).1(A:I0) (C7).4(B:I0) (C7).9(C:I0) (C7).12(D:I0)
ENTENS: (A5).3(A:O) (A6).9(C:I0) (B7).1(A:I0) (B7).4(B:I0) (B7).9(C:I0) (B7).12(D:I0)
F: (D7).15 (G8).1(A:I0)
G: (D7).14 (G7).9(C:I0)
GND: (D7).8 ; supply symbol labelled SUP ; also sheet 6,9,10
N$10: (A8).12(A:O) (G8).2(A:I1) (G8).11(C:I2)
N$33: (A7).3(A:O) (D7).7
N$35: (C6).1(CKB) (C6).12(QA) (C7).2(A:I1)
N$125: (B6).1(CKB) (B6).12(QA) (B7).2(A:I1)
N$126: (A5).8(C:O) (B5).13(B:I3)
N$127: (D8).1(A:I) (E7).6(B:O)
N$128: (B6).9(QB) (B7).5(B:I1)
N$129: (B6).8(QC) (B7).10(C:I1)
N$130: (B6).11(QD) (B7).13(D:I1)
N$131: (C5).2(A:I1) (C6).9(QB) (C7).5(B:I1)
N$133: (C6).8(QC) (C7).10(C:I1)
N$134: (C5).1(A:I0) (C6).11(QD) (C7).13(D:I1)
N$135: (A7).1(A:I0) (B7).3(A:O)
N$136: (A7).4(B:I0) (B7).6(B:O)
N$137: (A7).9(C:I0) (B7).8(C:O)
N$138: (A7).2(A:I1) (C7).3(A:O)
N$139: (A7).5(B:I1) (C7).6(B:O)
N$140: (A7).10(C:I1) (C7).8(C:O)
N$141: (A7).12(D:I0) (B7).11(D:O)
N$142: (A7).13(D:I1) (C7).11(D:O)
N$143: (A6).3(A:O) (C6).2(R0(1)) (C6).3(R0(2))
N$144: (A7).6(B:O) (D7).1
N$145: (A7).8(C:O) (D7).2
N$146: (A7).11(D:O) (D7).6
N$147: (F8).2(I1) (G8).12(A:O)
N$148: (F8).3(I2) (G8).8(C:O)
N$149: (F8).4(I3) (G8).6(B:O)
N$150: (F8).5(I4) (G7).12(A:O)
N$151: (F8).6(I5) (G7).6(B:O)
N$152: (F8).11(I6) (G7).8(C:O)
N$153: (E7).12(A:O) (F8).12(I7)
N$154: (D7).3 (D7).5 R40.1
N$156: (F8).1(I0) R41.1
N$163: (B8).3(A:I1) (C8).3(A:O)
N$170: (B8).1(A:O) (G7).2(A:I1) (G8).4(B:I1)
N$174: (A8).6(B:O) (G7).5(B:I2)
N$177: (D8).2(A:O) (E7).13(A:I2) (G7).11(C:I2)
N$211: (A5).11(D:O) (B5).5(A:I3)
ONES: (A5).4(B:I0) (B5).8(B:O)
SCORE: (F8).8(O) ; also sheet 8,9
SCOREEN: (A6).8(C:O) (D7).4
SCOREVEN: (A5).2(A:I1) (A5).5(B:I1) (C5).8(B:O)
START: (A6).1(A:I0) (B6).2(R0(1)) (B6).3(R0(2)) ; also sheet 6,8
TENS: (A5).1(A:I0) (B5).6(A:O)
VCC: (D7).16 R40.2 R41.2 ; also sheet 6,10
Unconnected: (A6).4(B:I0) (A6).5(B:I1) (A6).6(B:O) (A6).11(D:O) (A6).12(D:I0) (A6).13(D:I1) (A8).8(C:O) (A8).9(C:I0) (A8).10(C:I1) (A8).11(C:I2) (B8).4(B:O) (B8).5(B:I0) (B8).6(B:I1) (B8).8(C:I0) (B8).9(C:I1) (B8).10(C:O) (B8).11(D:I0) (B8).12(D:I1) (B8).13(D:O) (C8).4(B:I0) (C8).5(B:I1) (C8).6(B:O) (C8).8(C:O) (C8).9(C:I0) (C8).10(C:I1) (C8).11(D:O) (C8).12(D:I0) (C8).13(D:I1) (D8).3(B:I) (D8).4(B:O) (D8).5(C:I) (D8).6(C:O) (D8).8(D:O) (D8).9(D:I) (D8).10(E:O) (D8).11(E:I) (D8).12(F:O) (D8).13(F:I) (E7).8(C:O) (E7).9(C:I0) (E7).10(C:I1) (E7).11(C:I2)

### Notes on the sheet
- TENS place horizontal window
- Enables score 32px
  down from top of
  screen.
- Vertical position of score window...
- Enables ones score window
  to the right of the tens, with
  a 16 px gap between them.
- ONES place horizontal window
- Score Digit Windows are 32V x 16H
- Resets score.
- 7448
- Each of these letters corresponds
  to a segment in a 7 - Segment 
  display.
- Counting Tens
- Counting Ones
- Binary Coded Decimal 
  --to--
  7 - Segment Display
- Converting 7 - Segment from LED
  --to--
  Bars on the screen. (Like PONG)

## Sheet 8 of 10: Solder Points For Major Signals
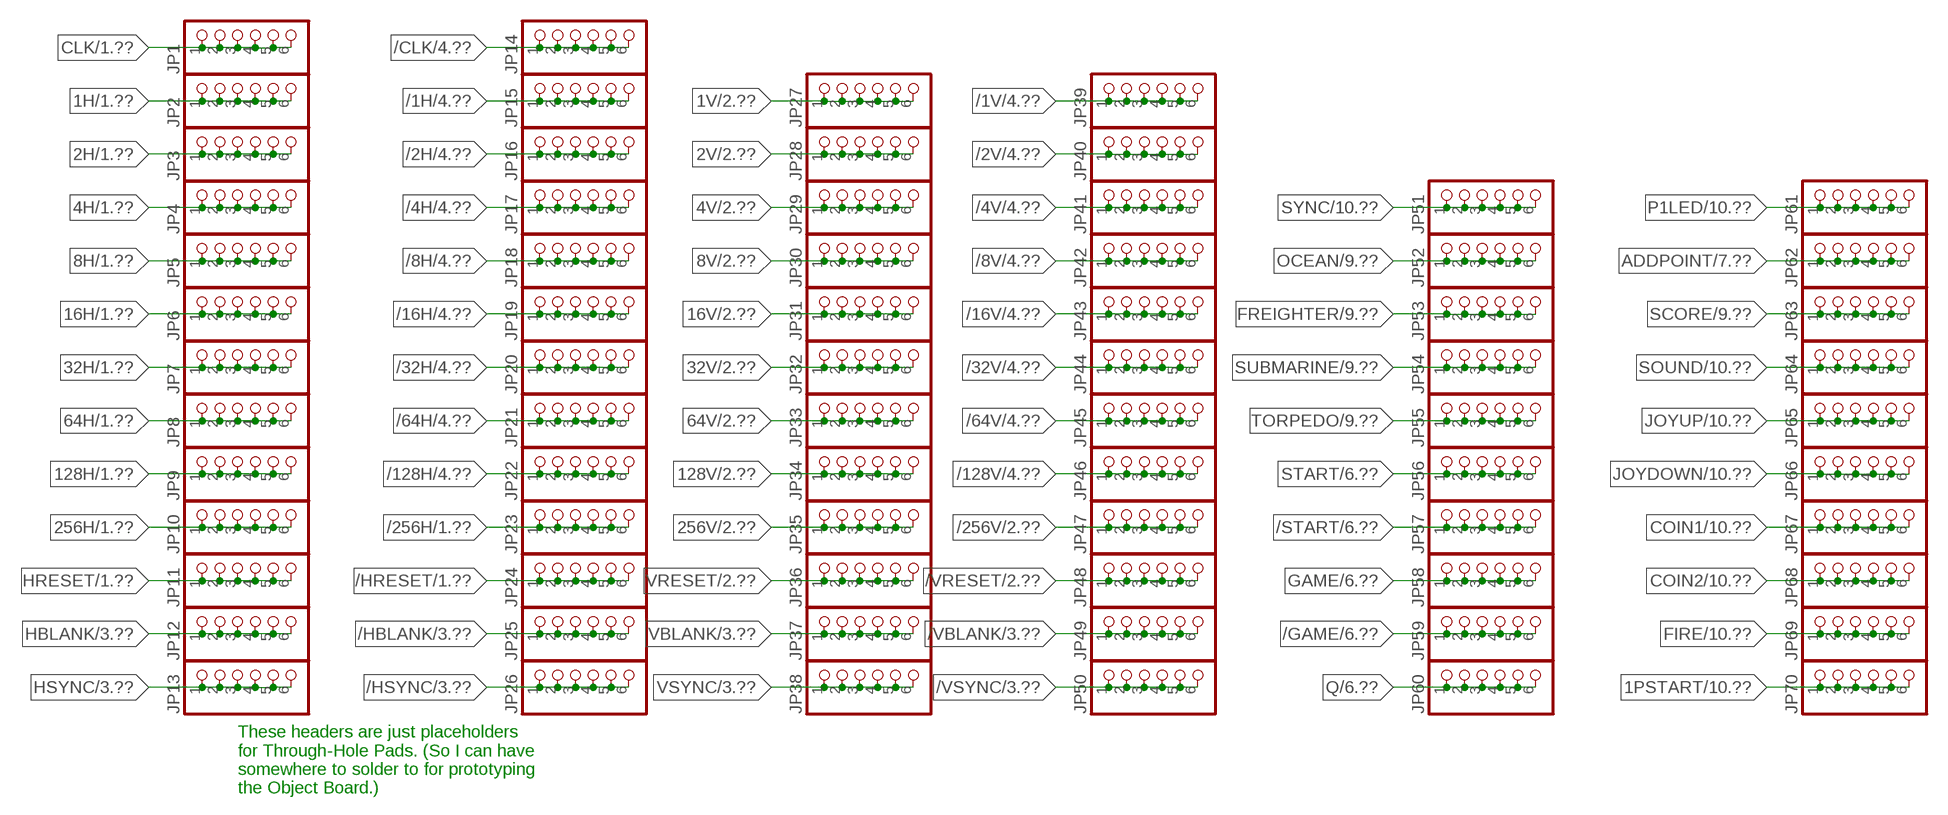
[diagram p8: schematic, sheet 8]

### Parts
JP1  PINHD-1X6  [1X06]
JP2  PINHD-1X6  [1X06]
JP3  PINHD-1X6  [1X06]
JP4  PINHD-1X6  [1X06]
JP5  PINHD-1X6  [1X06]
JP6  PINHD-1X6  [1X06]
JP7  PINHD-1X6  [1X06]
JP8  PINHD-1X6  [1X06]
JP9  PINHD-1X6  [1X06]
JP10  PINHD-1X6  [1X06]
JP11  PINHD-1X6  [1X06]
JP12  PINHD-1X6  [1X06]
JP13  PINHD-1X6  [1X06]
JP14  PINHD-1X6  [1X06]
JP15  PINHD-1X6  [1X06]
JP16  PINHD-1X6  [1X06]
JP17  PINHD-1X6  [1X06]
JP18  PINHD-1X6  [1X06]
JP19  PINHD-1X6  [1X06]
JP20  PINHD-1X6  [1X06]
JP21  PINHD-1X6  [1X06]
JP22  PINHD-1X6  [1X06]
JP23  PINHD-1X6  [1X06]
JP24  PINHD-1X6  [1X06]
JP25  PINHD-1X6  [1X06]
JP26  PINHD-1X6  [1X06]
JP27  PINHD-1X6  [1X06]
JP28  PINHD-1X6  [1X06]
JP29  PINHD-1X6  [1X06]
JP30  PINHD-1X6  [1X06]
JP31  PINHD-1X6  [1X06]
JP32  PINHD-1X6  [1X06]
JP33  PINHD-1X6  [1X06]
JP34  PINHD-1X6  [1X06]
JP35  PINHD-1X6  [1X06]
JP36  PINHD-1X6  [1X06]
JP37  PINHD-1X6  [1X06]
JP38  PINHD-1X6  [1X06]
JP39  PINHD-1X6  [1X06]
JP40  PINHD-1X6  [1X06]
JP41  PINHD-1X6  [1X06]
JP42  PINHD-1X6  [1X06]
JP43  PINHD-1X6  [1X06]
JP44  PINHD-1X6  [1X06]
JP45  PINHD-1X6  [1X06]
JP46  PINHD-1X6  [1X06]
JP47  PINHD-1X6  [1X06]
JP48  PINHD-1X6  [1X06]
JP49  PINHD-1X6  [1X06]
JP50  PINHD-1X6  [1X06]
JP51  PINHD-1X6  [1X06]
JP52  PINHD-1X6  [1X06]
JP53  PINHD-1X6  [1X06]
JP54  PINHD-1X6  [1X06]
JP55  PINHD-1X6  [1X06]
JP56  PINHD-1X6  [1X06]
JP57  PINHD-1X6  [1X06]
JP58  PINHD-1X6  [1X06]
JP59  PINHD-1X6  [1X06]
JP60  PINHD-1X6  [1X06]
JP61  PINHD-1X6  [1X06]
JP62  PINHD-1X6  [1X06]
JP63  PINHD-1X6  [1X06]
JP64  PINHD-1X6  [1X06]
JP65  PINHD-1X6  [1X06]
JP66  PINHD-1X6  [1X06]
JP67  PINHD-1X6  [1X06]
JP68  PINHD-1X6  [1X06]
JP69  PINHD-1X6  [1X06]
JP70  PINHD-1X6  [1X06]

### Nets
1H: JP2.1 JP2.2 JP2.3 JP2.4 JP2.5 JP2.6 ; also sheet 1,4
1PSTART: JP70.1 JP70.2 JP70.3 JP70.4 JP70.5 JP70.6 ; also sheet 6,10
1V: JP27.1 JP27.2 JP27.3 JP27.4 JP27.5 JP27.6 ; also sheet 2,4
2H: JP3.1 JP3.2 JP3.3 JP3.4 JP3.5 JP3.6 ; also sheet 1,4,5
2V: JP28.1 JP28.2 JP28.3 JP28.4 JP28.5 JP28.6 ; also sheet 2,4
4H: JP4.1 JP4.2 JP4.3 JP4.4 JP4.5 JP4.6 ; also sheet 1,4,7
4V: JP29.1 JP29.2 JP29.3 JP29.4 JP29.5 JP29.6 ; also sheet 2,3,4,7
8H: JP5.1 JP5.2 JP5.3 JP5.4 JP5.5 JP5.6 ; also sheet 1,4,7
8V: JP30.1 JP30.2 JP30.3 JP30.4 JP30.5 JP30.6 ; also sheet 2,3,4,7
16H: JP6.1 JP6.2 JP6.3 JP6.4 JP6.5 JP6.6 ; also sheet 1,3,4,7
16V: JP31.1 JP31.2 JP31.3 JP31.4 JP31.5 JP31.6 ; also sheet 2,3,4,7
32H: JP7.1 JP7.2 JP7.3 JP7.4 JP7.5 JP7.6 ; also sheet 1,3,4,7
32V: JP32.1 JP32.2 JP32.3 JP32.4 JP32.5 JP32.6 ; also sheet 2,4,7
64H: JP8.1 JP8.2 JP8.3 JP8.4 JP8.5 JP8.6 ; also sheet 1,3,4,7
64V: JP33.1 JP33.2 JP33.3 JP33.4 JP33.5 JP33.6 ; also sheet 2,4
128H: JP9.1 JP9.2 JP9.3 JP9.4 JP9.5 JP9.6 ; also sheet 1,4,7
128V: JP34.1 JP34.2 JP34.3 JP34.4 JP34.5 JP34.6 ; also sheet 2,4,5,6
256H: JP10.1 JP10.2 JP10.3 JP10.4 JP10.5 JP10.6 ; also sheet 1,7
256V: JP35.1 JP35.2 JP35.3 JP35.4 JP35.5 JP35.6 ; also sheet 2,6
/1H: JP15.1 JP15.2 JP15.3 JP15.4 JP15.5 JP15.6 ; also sheet 4
/1V: JP39.1 JP39.2 JP39.3 JP39.4 JP39.5 JP39.6 ; also sheet 4,5
/2H: JP16.1 JP16.2 JP16.3 JP16.4 JP16.5 JP16.6 ; also sheet 4
/2V: JP40.1 JP40.2 JP40.3 JP40.4 JP40.5 JP40.6 ; also sheet 4,5
/4H: JP17.1 JP17.2 JP17.3 JP17.4 JP17.5 JP17.6 ; also sheet 4
/4V: JP41.1 JP41.2 JP41.3 JP41.4 JP41.5 JP41.6 ; also sheet 4,5
/8H: JP18.1 JP18.2 JP18.3 JP18.4 JP18.5 JP18.6 ; also sheet 4
/8V: JP42.1 JP42.2 JP42.3 JP42.4 JP42.5 JP42.6 ; also sheet 4,5
/16H: JP19.1 JP19.2 JP19.3 JP19.4 JP19.5 JP19.6 ; also sheet 4,7
/16V: JP43.1 JP43.2 JP43.3 JP43.4 JP43.5 JP43.6 ; also sheet 4,5,7
/32H: JP20.1 JP20.2 JP20.3 JP20.4 JP20.5 JP20.6 ; also sheet 4,7
/32V: JP44.1 JP44.2 JP44.3 JP44.4 JP44.5 JP44.6 ; also sheet 4,5
/64H: JP21.1 JP21.2 JP21.3 JP21.4 JP21.5 JP21.6 ; also sheet 4,7
/64V: JP45.1 JP45.2 JP45.3 JP45.4 JP45.5 JP45.6 ; also sheet 4,5,7
/128H: JP22.1 JP22.2 JP22.3 JP22.4 JP22.5 JP22.6 ; also sheet 4,7
/128V: JP46.1 JP46.2 JP46.3 JP46.4 JP46.5 JP46.6 ; also sheet 4,7
/256H: JP23.1 JP23.2 JP23.3 JP23.4 JP23.5 JP23.6 ; also sheet 1,7
/256V: JP47.1 JP47.2 JP47.3 JP47.4 JP47.5 JP47.6 ; also sheet 2,7
/CLK: JP14.1 JP14.2 JP14.3 JP14.4 JP14.5 JP14.6 ; also sheet 4
/GAME: JP59.1 JP59.2 JP59.3 JP59.4 JP59.5 JP59.6 ; also sheet 6
/HBLANK: JP25.1 JP25.2 JP25.3 JP25.4 JP25.5 JP25.6 ; also sheet 3
/HRESET: JP24.1 JP24.2 JP24.3 JP24.4 JP24.5 JP24.6 ; also sheet 1,3
/HSYNC: JP26.1 JP26.2 JP26.3 JP26.4 JP26.5 JP26.6 ; also sheet 3
/START: JP57.1 JP57.2 JP57.3 JP57.4 JP57.5 JP57.6 ; also sheet 6
/VBLANK: JP49.1 JP49.2 JP49.3 JP49.4 JP49.5 JP49.6 ; also sheet 3
/VRESET: JP48.1 JP48.2 JP48.3 JP48.4 JP48.5 JP48.6 ; also sheet 2
/VSYNC: JP50.1 JP50.2 JP50.3 JP50.4 JP50.5 JP50.6 ; also sheet 3
ADDPOINT: JP62.1 JP62.2 JP62.3 JP62.4 JP62.5 JP62.6 ; also sheet 7
CLK: JP1.1 JP1.2 JP1.3 JP1.4 JP1.5 JP1.6 ; also sheet 1,4
COIN1: JP67.1 JP67.2 JP67.3 JP67.4 JP67.5 JP67.6 ; also sheet 6,10
COIN2: JP68.1 JP68.2 JP68.3 JP68.4 JP68.5 JP68.6 ; also sheet 6,10
FIRE: JP69.1 JP69.2 JP69.3 JP69.4 JP69.5 JP69.6 ; also sheet 10
FREIGHTER: JP53.1 JP53.2 JP53.3 JP53.4 JP53.5 JP53.6 ; also sheet 9
GAME: JP58.1 JP58.2 JP58.3 JP58.4 JP58.5 JP58.6 ; also sheet 6
HBLANK: JP12.1 JP12.2 JP12.3 JP12.4 JP12.5 JP12.6 ; also sheet 3
HRESET: JP11.1 JP11.2 JP11.3 JP11.4 JP11.5 JP11.6 ; also sheet 1,2
HSYNC: JP13.1 JP13.2 JP13.3 JP13.4 JP13.5 JP13.6 ; also sheet 3
JOYDOWN: JP66.1 JP66.2 JP66.3 JP66.4 JP66.5 JP66.6 ; also sheet 10
JOYUP: JP65.1 JP65.2 JP65.3 JP65.4 JP65.5 JP65.6 ; also sheet 10
OCEAN: JP52.1 JP52.2 JP52.3 JP52.4 JP52.5 JP52.6 ; also sheet 5,9
P1LED: JP61.1 JP61.2 JP61.3 JP61.4 JP61.5 JP61.6 ; also sheet 6,10
Q: JP60.1 JP60.2 JP60.3 JP60.4 JP60.5 JP60.6 ; also sheet 6
SCORE: JP63.1 JP63.2 JP63.3 JP63.4 JP63.5 JP63.6 ; also sheet 7,9
SOUND: JP64.1 JP64.2 JP64.3 JP64.4 JP64.5 JP64.6 ; also sheet 10
START: JP56.1 JP56.2 JP56.3 JP56.4 JP56.5 JP56.6 ; also sheet 6,7
SUBMARINE: JP54.1 JP54.2 JP54.3 JP54.4 JP54.5 JP54.6 ; also sheet 9
SYNC: JP51.1 JP51.2 JP51.3 JP51.4 JP51.5 JP51.6 ; also sheet 3,10
TORPEDO: JP55.1 JP55.2 JP55.3 JP55.4 JP55.5 JP55.6 ; also sheet 9
VBLANK: JP37.1 JP37.2 JP37.3 JP37.4 JP37.5 JP37.6 ; also sheet 3
VRESET: JP36.1 JP36.2 JP36.3 JP36.4 JP36.5 JP36.6 ; also sheet 2,3
VSYNC: JP38.1 JP38.2 JP38.3 JP38.4 JP38.5 JP38.6 ; also sheet 3

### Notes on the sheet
- These headers are just placeholders
  for Through-Hole Pads. (So I can have
  somewhere to solder to for prototyping
  the Object Board.)

## Sheet 9 of 10: RGB Out
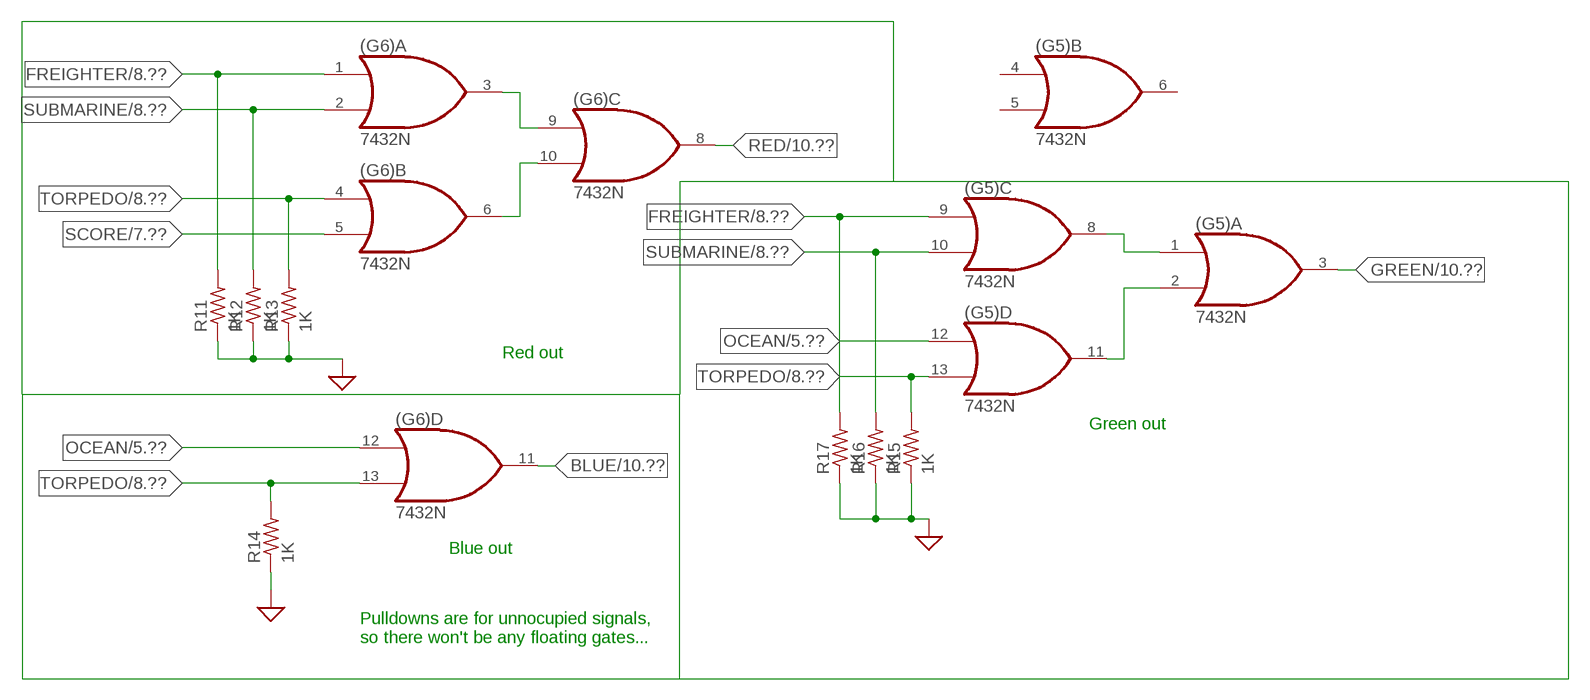
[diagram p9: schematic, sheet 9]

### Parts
(G5)  7432N  [DIL14]
(G6)  7432N  [DIL14]
R11  1K  R-US_0207/10  [0207/10]
R12  1K  R-US_0207/10  [0207/10]
R13  1K  R-US_0207/10  [0207/10]
R14  1K  R-US_0207/10  [0207/10]
R15  1K  R-US_0207/10  [0207/10]
R16  1K  R-US_0207/10  [0207/10]
R17  1K  R-US_0207/10  [0207/10]

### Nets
BLUE: (G6).11(D:O) ; also sheet 10
FREIGHTER: (G5).9(C:I0) (G6).1(A:I0) R11.2 R17.2 ; also sheet 8
GND: R11.1 R12.1 R13.1 R14.1 R15.1 R16.1 R17.1 ; supply symbol labelled SUP ; also sheet 6,7,10
GREEN: (G5).3(A:O) ; also sheet 10
N$115: (G6).3(A:O) (G6).9(C:I0)
N$117: (G6).6(B:O) (G6).10(C:I1)
N$121: (G5).2(A:I1) (G5).11(D:O)
N$122: (G5).1(A:I0) (G5).8(C:O)
OCEAN: (G5).12(D:I0) (G6).12(D:I0) ; also sheet 5,8
RED: (G6).8(C:O) ; also sheet 10
SCORE: (G6).5(B:I1) ; also sheet 7,8
SUBMARINE: (G5).10(C:I1) (G6).2(A:I1) R12.2 R16.2 ; also sheet 8
TORPEDO: (G5).13(D:I1) (G6).4(B:I0) (G6).13(D:I1) R13.2 R14.2 R15.2 ; also sheet 8
Unconnected: (G5).4(B:I0) (G5).5(B:I1) (G5).6(B:O)

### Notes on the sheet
- Red out
- Green out
- Blue out
- Pulldowns are for unnocupied signals,
  so there won't be any floating gates...

## Sheet 10 of 10: Card Edge Connector
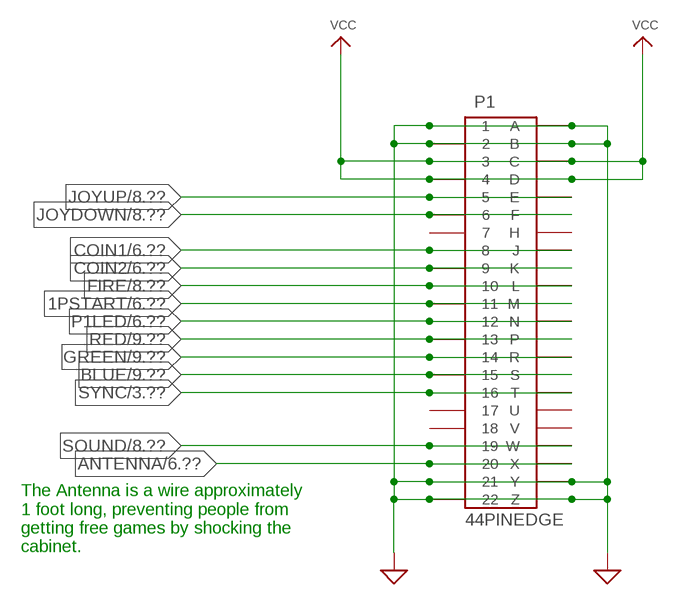
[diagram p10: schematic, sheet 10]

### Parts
P1  44PINEDGE  [44PINEDGE]

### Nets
1PSTART: P1.11 P1.M ; also sheet 6,8
ANTENNA: P1.20 P1.X ; also sheet 6
BLUE: P1.15 P1.S ; also sheet 9
COIN1: P1.8 P1.J ; also sheet 6,8
COIN2: P1.9 P1.K ; also sheet 6,8
FIRE: P1.10 P1.L ; also sheet 8
GND: P1.1 P1.2 P1.21 P1.22 P1.A P1.B P1.Y P1.Z ; supply symbol labelled SUP ; also sheet 6,7,9
GREEN: P1.14 P1.R ; also sheet 9
JOYDOWN: P1.6 P1.F ; also sheet 8
JOYUP: P1.5 P1.E ; also sheet 8
P1LED: P1.12 P1.N ; also sheet 6,8
RED: P1.13 P1.P ; also sheet 9
SOUND: P1.19 P1.W ; also sheet 8
SYNC: P1.16 P1.T ; also sheet 3,8
VCC: P1.3 P1.4 P1.C P1.D ; also sheet 6,7
Unconnected: P1.7 P1.17 P1.18 P1.H P1.U P1.V

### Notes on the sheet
- The Antenna is a wire approximately
  1 foot long, preventing people from
  getting free games by shocking the
  cabinet.

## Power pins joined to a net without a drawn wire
GND: (A1).7(P:GND) (A2).7(P:GND) (A3).7(P:GND) (A4).7(P:GND) (A5).7(P:GND) (A6).7(P:GND) (A7).7(P:GND) (A8).7(P:GND) (B1).7(P:GND) (B2).7(P:GND) (B3).7(P:GND) (B4).7(P:GND) (B5).7(P:GND) (B6).10(GND) (B7).7(P:GND) (B8).7(P:GND) (C1).10(GND) (C2).10(GND) (C3).7(P:GND) (C4).7(P:GND) (C5).7(P:GND) (C6).10(GND) (C7).7(P:GND) (C8).7(P:GND) (D1).10(GND) (D2).7(GND) (D3).7(P:GND) (D4).7(P:GND) (D6).7(P:GND) (D8).7(P:GND) (E1).10(GND) (E2).7(P:GND) (E3).7(P:GND) (E4).7(P:GND) (E5).7(P:GND) (E6).7(P:GND) (E7).7(P:GND) (F1).7(P:GND) (F2).7(P:GND) (F3).7(GND) (F4).7(P:GND) (F5).7(P:GND) (F6).7(P:GND) (F7).7(P:GND) (F8).7(GND) (G5).7(P:GND) (G6).7(P:GND) (G7).7(P:GND) (G8).7(P:GND)
VCC: (A1).14(P:VCC) (A2).14(P:VCC) (A3).14(P:VCC) (A4).14(P:VCC) (A5).14(P:VCC) (A6).14(P:VCC) (A7).14(P:VCC) (A8).14(P:VCC) (B1).14(P:VCC) (B2).14(P:VCC) (B3).14(P:VCC) (B4).14(P:VCC) (B5).14(P:VCC) (B6).5(VCC) (B7).14(P:VCC) (B8).14(P:VCC) (C1).5(VCC) (C2).5(VCC) (C3).14(P:VCC) (C4).14(P:VCC) (C5).14(P:VCC) (C6).5(VCC) (C7).14(P:VCC) (C8).14(P:VCC) (D1).5(VCC) (D2).14(VCC) (D3).14(P:VCC) (D4).14(P:VCC) (D6).14(P:VCC) (D8).14(P:VCC) (E1).5(VCC) (E2).14(P:VCC) (E3).14(P:VCC) (E4).14(P:VCC) (E5).14(P:VCC) (E6).14(P:VCC) (E7).14(P:VCC) (F1).14(P:VCC) (F2).14(P:VCC) (F3).14(VCC) (F4).14(P:VCC) (F5).14(P:VCC) (F6).14(P:VCC) (F7).14(P:VCC) (F8).14(VCC) (G5).14(P:VCC) (G6).14(P:VCC) (G7).14(P:VCC) (G8).14(P:VCC)

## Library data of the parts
(A1) (B4) (C4) (D4) (D6) (D8) (E3) (F1) (F5) = 74xx-us:74*04: Hex INVERTER
(A2) (B8) = 74xx-us:74*02: Quad 2-input NOR gate
(A3) (C8) (F2) = 74xx-us:74*00: Quad 2-input NAND gate
(A4) (B2) (E7) (G7) (G8) = 74xx-us:74*10: Triple 3-input NAND gate
(A5) (B7) (C7) (E4) (E5) = 74xx-us:74*08: Quad 2-input AND gate
(A6) (A7) (F4) (G5) (G6) = 74xx-us:74*32: Quad 2-input OR gate
(A8) = 74xx-us:74*27: Triple 3-input NOR gate
(B1) = 74xx-us:74*86: Quad 2-input EXCLUSIV-OR (XOR) gate
(B3) (D3) (E6) (F6) (F7) = 74xx-us:74*74: Dual D type positive edge triggered FLIP FLOP, preset and clear
(B5) (C5) = 74xx-us:74*21: Dual 4-input AND gate
(B6) (C1) (C2) (C6) (D1) (E1) = 74xx-us:74*93: Decade, divide by twelve and binary COUNTER
(C3) (E2) = 74xx-us:74*107: Dual J-K FLIP FLOP, clear
(D2) (F3) (F8) = 74xx-us:74*30: 8-input NAND gate
(D5) = SparkFun-IC-Special-Function:555: General purpose bipolar Timer Datasheet SparkFun Products SparkFun SparkPunk Sequencer Kit (KIT-12707) Storefront Component: 555 Timer (COM-09273) Two parts valid for production: VFP: IC-11930 (M7555 PTH) VFP: IC-09173 (555 PTH) - Preferred; PROD_ID: IC-09173; PROD_ID_ALT: IC-09173
(D7) = ic-package:DIL16: Dual In Line / Socket
C1 C2 = rcl:C-US: CAPACITOR, American symbol
C4-C7 = adafruit:C-US: CAPACITOR, American symbol
D1 D3-D5 = adafruit:1N4004: DIODE
JP1-JP70 = adafruit:PINHD-1X6: PIN HEADER
P1 = edge-156:44PINEDGE: 44 PIN EDGE CONNECTOR FOR PCB
Q1 = special:XTAL/S: CRYSTAL
Q2 = adafruit:2N2907*: PNP Transistor Big Oval pads
R1-R4 R6-R8 = rcl:R-US_: RESISTOR, American symbol
R5 R9-R17 R28-R35 R37 R38 R40 R41 R47 = adafruit:R-US_: RESISTOR, American symbol
SW1 = adafruit:SWITCH_PUSHBUTTON: Buttons
T1 T2 = adafruit:2N2222: NPN TRANSISTOR Big oval pads
VR1 = SparkFun-Resistors:TRIMPOT: Trimming Potentiometer (Trimpot) Three-terminal potentiometers, with an adjustable wiper and two adjustable resistors. A pot can be used to create a configurable voltage divider, or as a variable resistor. "Trimpots" are a subset of potentiometers, usually intended for "set-and-forget"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; PROD_ID: RES-09730; SF_SKU: COM-09806; VALUE: 10k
